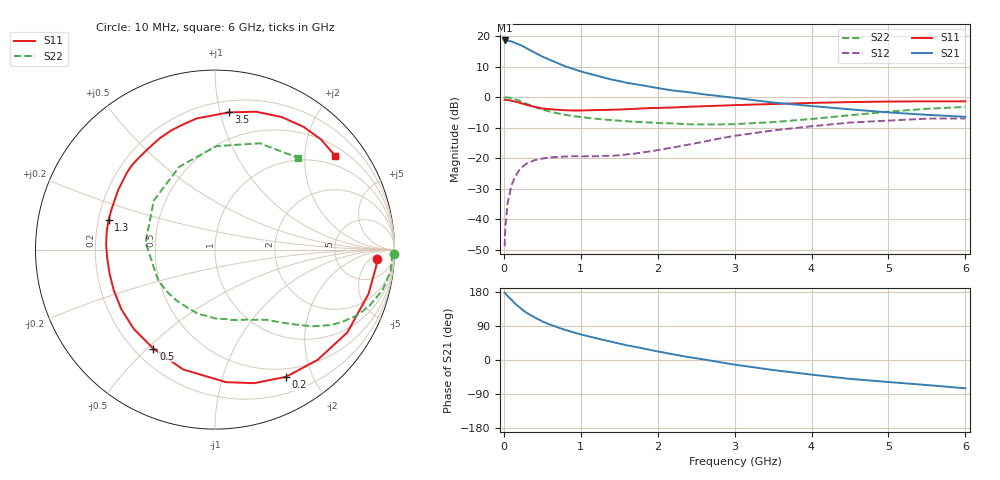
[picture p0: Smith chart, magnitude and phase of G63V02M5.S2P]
! SIEMENS Small Signal Semiconductors
! BFG193
! Si NPN RF Bipolar Junction Transistor in SOT223
! VCE = 3 V  IC = 2.5 mA
! Common Emitter S-Parameters:  August  1996
# GHz  S  MA  R  50
!  f  S11  S21  S12  S22
! GHz  MAG  ANG  MAG  ANG  MAG  ANG  MAG  ANG
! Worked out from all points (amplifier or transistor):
!   36 points, 10 MHz to 6 GHz, reference 50 ohm
!   highest |S21| = 18.5 dB at 10 MHz (marker M1)
!   |S21| within 3 dB of that: start of sweep to 327.4 MHz
!   unconditionally stable (mu >= 1): 1.317 GHz to 2.586 GHz
!   at 250 MHz: K = 0.21, MSG = 19.6 dB, |S12| = -22.7 dB
!   at 1.4 GHz: K = 1.07, MAG = 10.9 dB, |S12| = -19.3 dB
!   at 6 GHz: K = 0.94, MSG = 0.3 dB, |S12| = -7.0 dB
!   S11 on the Smith chart (normalised r, x): 10 MHz: 15, -9; 200 MHz: 0.39, -1.63; 500 MHz: 0.27, -0.52; 1.3 GHz: 0.24, +0.13; 3.5 GHz: 0.28, +1.06; 6 GHz: 0.72, +2.73
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0.01  0.9062 -3.3  8.461 177.6  0.0036 90.6  0.996 -1.5
0.02  0.9017 -6.4  8.458 176.3  0.0076 86.2  0.9869 -2.8
0.05  0.8903 -16.1  8.374 168.3  0.0185 80.6  0.986 -7.1
0.1  0.87 -32.0  8.125 159.1  0.0361 73.5  0.9598 -13.7
0.15  0.8393 -47.0  7.651 148.0  0.0509 64.3  0.9162 -19.9
0.2  0.812 -60.8  7.257 139.7  0.0632 58.0  0.8719 -24.9
0.25  0.7753 -73.7  6.777 131.3  0.0736 51.7  0.8172 -29.4
0.3  0.7412 -85.2  6.245 124.1  0.0816 47.1  0.7739 -32.9
0.4  0.6911 -104.9  5.362 112.6  0.0922 39.0  0.6894 -38.3
0.5  0.6497 -121.9  4.601 101.9  0.0982 32.8  0.6245 -42.2
0.6  0.6325 -135.7  4.055 93.5  0.1024 29.2  0.5775 -45.4
0.7  0.6186 -147.5  3.594 86.1  0.1048 26.6  0.5412 -48.4
0.8  0.6079 -158.1  3.194 79.3  0.106 24.5  0.5103 -51.1
1.1  0.607 177.5  2.426 62.4  0.1069 22.8  0.4541 -59.5
1.3  0.6155 164.4  2.089 52.7  0.1087 23.9  0.428 -65.6
1.6  0.6338 148.1  1.71 38.7  0.1148 27.1  0.4023 -76.9
2.2  0.675 123.4  1.278 15.0  0.1491 31.8  0.3704 -104.4
2.8  0.7217 103.5  1.039 -5.5  0.2085 27.8  0.3559 -139.4
3.5  0.7683 84.3  0.813 -26.4  0.2839 13.7  0.3887 174.0
4.5  0.8268 63.3  0.629 -49.8  0.3819 -9.4  0.5029 113.3
5.5  0.8517 46.2  0.511 -66.1  0.4428 -37.3  0.6425 67.2
6  0.8493 38.1  0.475 -74.7  0.4455 -52.4  0.6889 48.1
